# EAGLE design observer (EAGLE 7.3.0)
AUTHOR: B. Campbell, N. Jackson, C. Kreng, A. Zhen; REV: D; TITLE: Observer

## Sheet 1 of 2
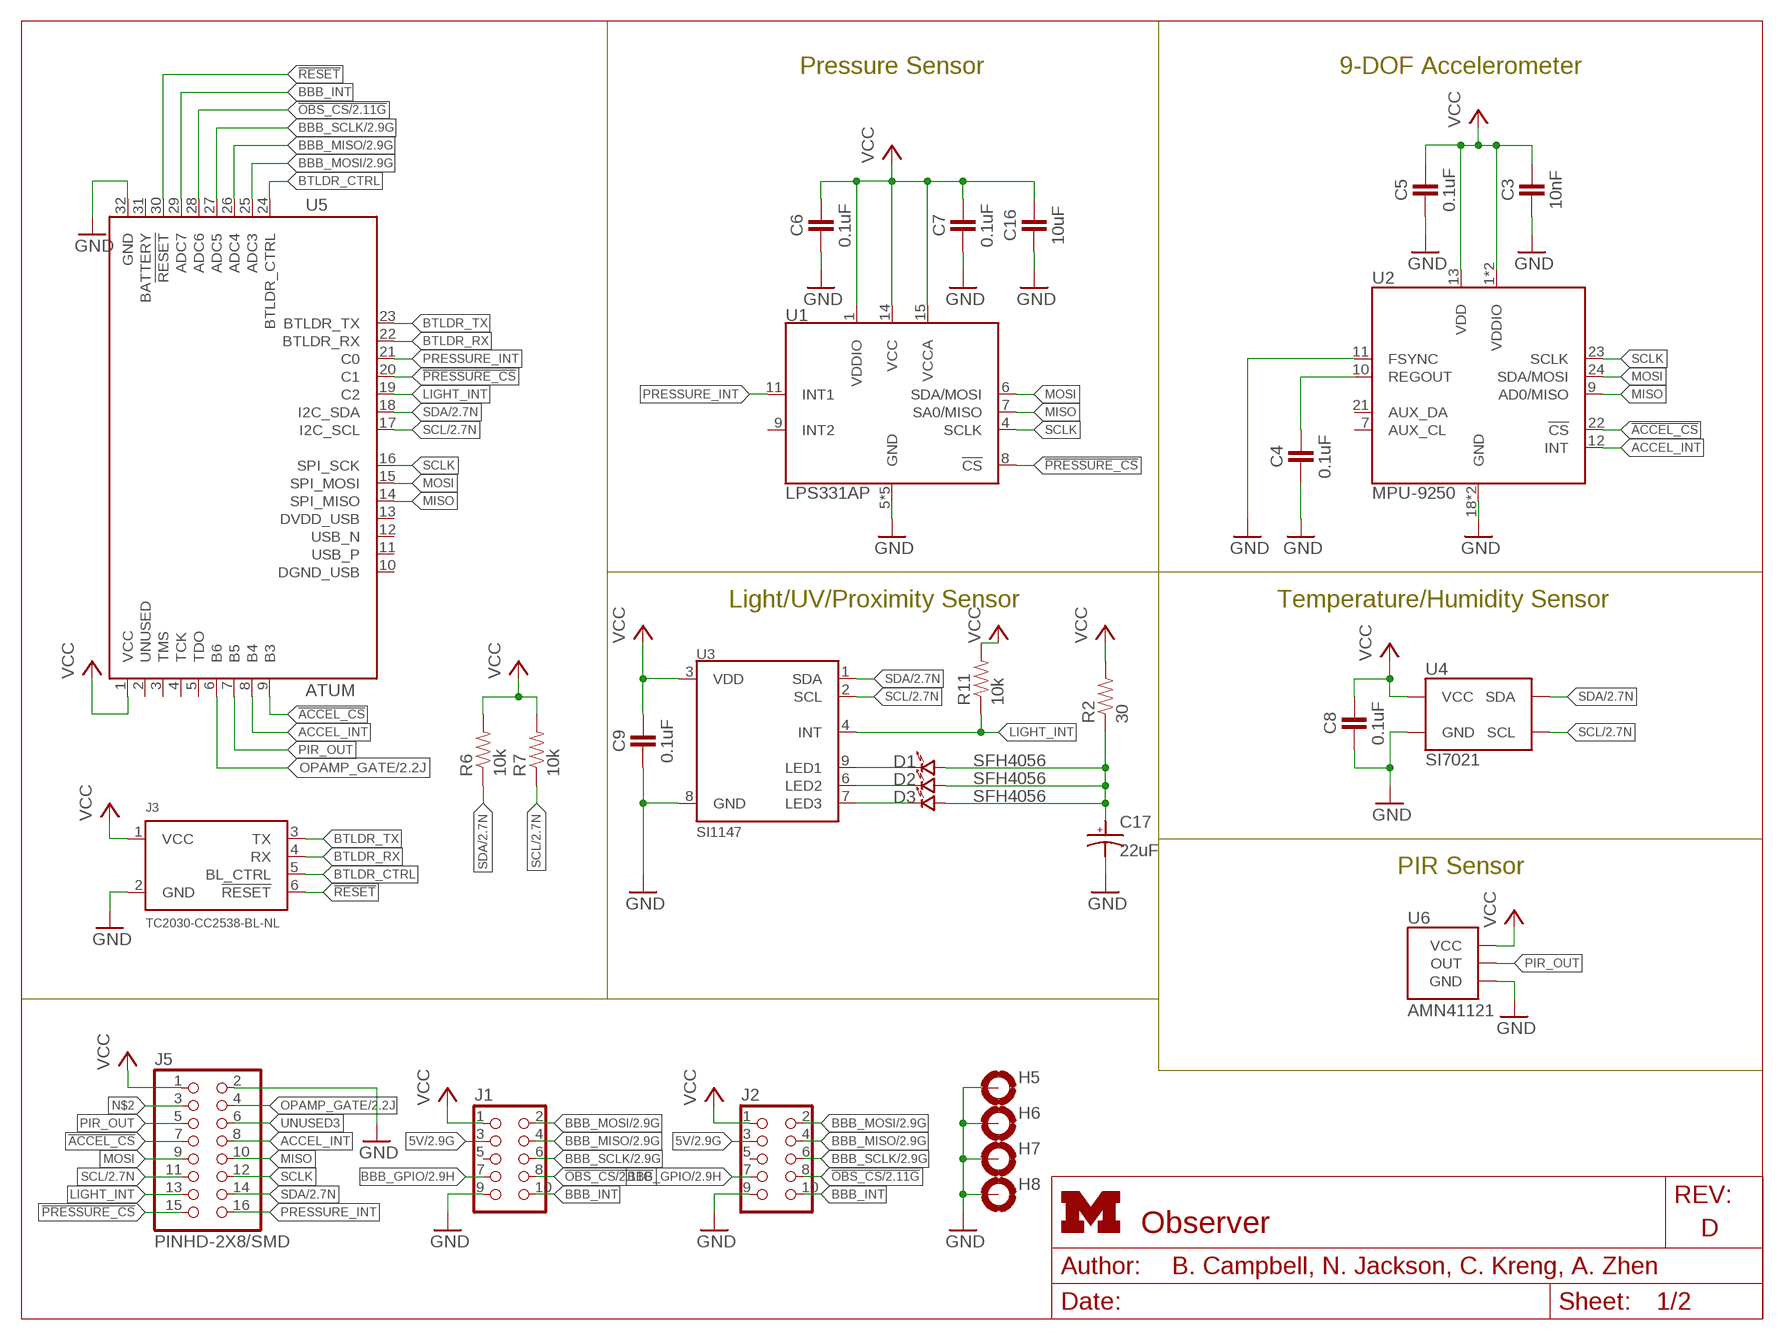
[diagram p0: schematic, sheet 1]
FRAME1 (LETTER_L): HEIGHT: 8.5in; WIDTH: 11in

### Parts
C3  10nF  CAPACITOR  [0402_CAP]
C4  0.1uF  CAPACITOR  [0402_CAP]
C5  0.1uF  CAPACITOR  [0402_CAP]
C6  0.1uF  CAPACITOR  [0402_CAP]
C7  0.1uF  CAPACITOR  [0402_CAP]
C8  0.1uF  CAPACITOR  [0402_CAP]
C9  0.1uF  CAPACITOR  [0402_CAP]
C16  10uF  CAPACITOR  [0402_CAP]
C17  22uF  CAP_POL0603  [CAP0603]
D1  SFH4056  [SFH4056]
D2  SFH4056  [SFH4056]
D3  SFH4056  [SFH4056]
H5  MOUNT-PAD-ROUND3.2  [3,2-PAD]
H6  MOUNT-PAD-ROUND3.2  [3,2-PAD]
H7  MOUNT-PAD-ROUND3.2  [3,2-PAD]
H8  MOUNT-PAD-ROUND3.2  [3,2-PAD]
J1  CON_HEADER_2X05-SMD+SHROUDED  [PINSHRD_SMT_2X05]
J2  CON_HEADER_2X05-SMD+SHROUDED  [PINSHRD_SMT_2X05]
J3  TC2030-CC2538-BL-NL  [TC2030-IDC-NL]
J5  PINHD-2X8/SMD  [2X8/SMD]
R2  30  RESISTOR0402_RES  [0402_RES]
R6  10k  RESISTOR0402_RES  [0402_RES]
R7  10k  RESISTOR0402_RES  [0402_RES]
R11  10k  RESISTOR0402_RES  [0402_RES]
U1  LPS331AP  [HCLGA-16/3MM]
U2  MPU-9250  [QFN-24/3MM]
U3  SI1147  [QFN-10/2MM]
U4  SI7021  [DFN-6/3MM]
U5  ATUM  [ATUM]
U6  AMN41121  [AMN2]

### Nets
5V: J1.3 J2.3 ; also sheet 2
!ACCEL_CS: J5.7 U2.22(!CS) U5.9(B3)
!OBS_CS: J1.8 J2.8 U5.28(ADC6) ; also sheet 2
!PRESSURE_CS: J5.15 U1.8(!CS) U5.20(C1)
!RESET: J3.6(!RESET) U5.30(!RESET)
ACCEL_INT: J5.8 U2.12(INT) U5.8(B4)
BBB_GPIO: J1.7 J2.7 ; also sheet 2
BBB_INT: J1.10 J2.10 U5.29(ADC7)
BBB_MISO: J1.4 J2.4 U5.26(ADC4) ; also sheet 2
BBB_MOSI: J1.2 J2.2 U5.25(ADC3) ; also sheet 2
BBB_SCLK: J1.6 J2.6 U5.27(ADC5) ; also sheet 2
BTLDR_CTRL: J3.5(BL_CTRL) U5.24(BTLDR_CTRL)
BTLDR_RX: J3.4(RX) U5.22(BTLDR_RX)
BTLDR_TX: J3.3(TX) U5.23(BTLDR_TX)
GND: C3.2 C4.2 C5.2 C6.2 C7.2 C8.2 C9.2 C16.2 C17.NEG(ANODE) H5.B3,2(MOUNT) H6.B3,2(MOUNT) H7.B3,2(MOUNT) H8.B3,2(MOUNT) J1.9 J2.9 J3.2(GND) J5.2 U1.5(GND) U1.10(GND) U1.12(GND) U1.13(GND) U1.16(GND) U2.11(FSYNC) U2.18(GND) U2.20(GND) U3.8(GND) U4.2(GND) U5.32(GND) U6.GND ; also sheet 2
LIGHT_INT: J5.13 R11.1 U3.4(INT) U5.19(C2)
MISO: J5.10 U1.7(SA0/MISO) U2.9(AD0/MISO) U5.14(SPI_MISO)
MOSI: J5.9 U1.6(SDA/MOSI) U2.24(SDA/MOSI) U5.15(SPI_MOSI)
N$2: J5.3
N$3: C4.1 U2.10(REGOUT)
N$4: D1.CATHODE U3.9(LED1)
N$6: D2.CATHODE U3.6(LED2)
N$7: D3.CATHODE U3.7(LED3)
N$8: C17.POS(CATHODE) D1.ANODE D2.ANODE D3.ANODE R2.1
OPAMP_GATE: J5.4 U5.6(B6) ; also sheet 2
PIR_OUT: J5.5 U5.7(B5) U6.OUT
PRESSURE_INT: J5.16 U1.11(INT1) U5.21(C0)
SCL: J5.11 R7.1 U3.2(SCL) U4.6(SCL) U5.17(I2C_SCL) ; also sheet 2
SCLK: J5.12 U1.4(SCLK) U2.23(SCLK) U5.16(SPI_SCK)
SDA: J5.14 R6.1 U3.1(SDA) U4.1(SDA) U5.18(I2C_SDA) ; also sheet 2
UNUSED3: J5.6
VCC: C3.1 C5.1 C6.1 C7.1 C8.1 C9.1 C16.1 J1.1 J2.1 J3.1(VCC) J5.1 R2.2 R6.2 R7.2 R11.2 U1.1(VDDIO) U1.14(VCC) U1.15(VCCA) U2.1(VDDIO) U2.8(VDDIO) U2.13(VDD) U3.3(VDD) U4.5(VCC) U5.1(VCC) U6.VCC ; also sheet 2
Unconnected: J1.5 J2.5 U1.9(INT2) U2.7(AUX_CL) U2.21(AUX_DA) U5.2(UNUSED) U5.3(TMS) U5.4(TCK) U5.5(TDO) U5.10(DGND_USB) U5.11(USB_P) U5.12(USB_N) U5.13(DVDD_USB) U5.31(BATTERY)

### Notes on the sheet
- Pressure Sensor | 9-DOF Accelerometer
- Light/UV/Proximity Sensor | Temperature/Humidity Sensor
- PIR Sensor

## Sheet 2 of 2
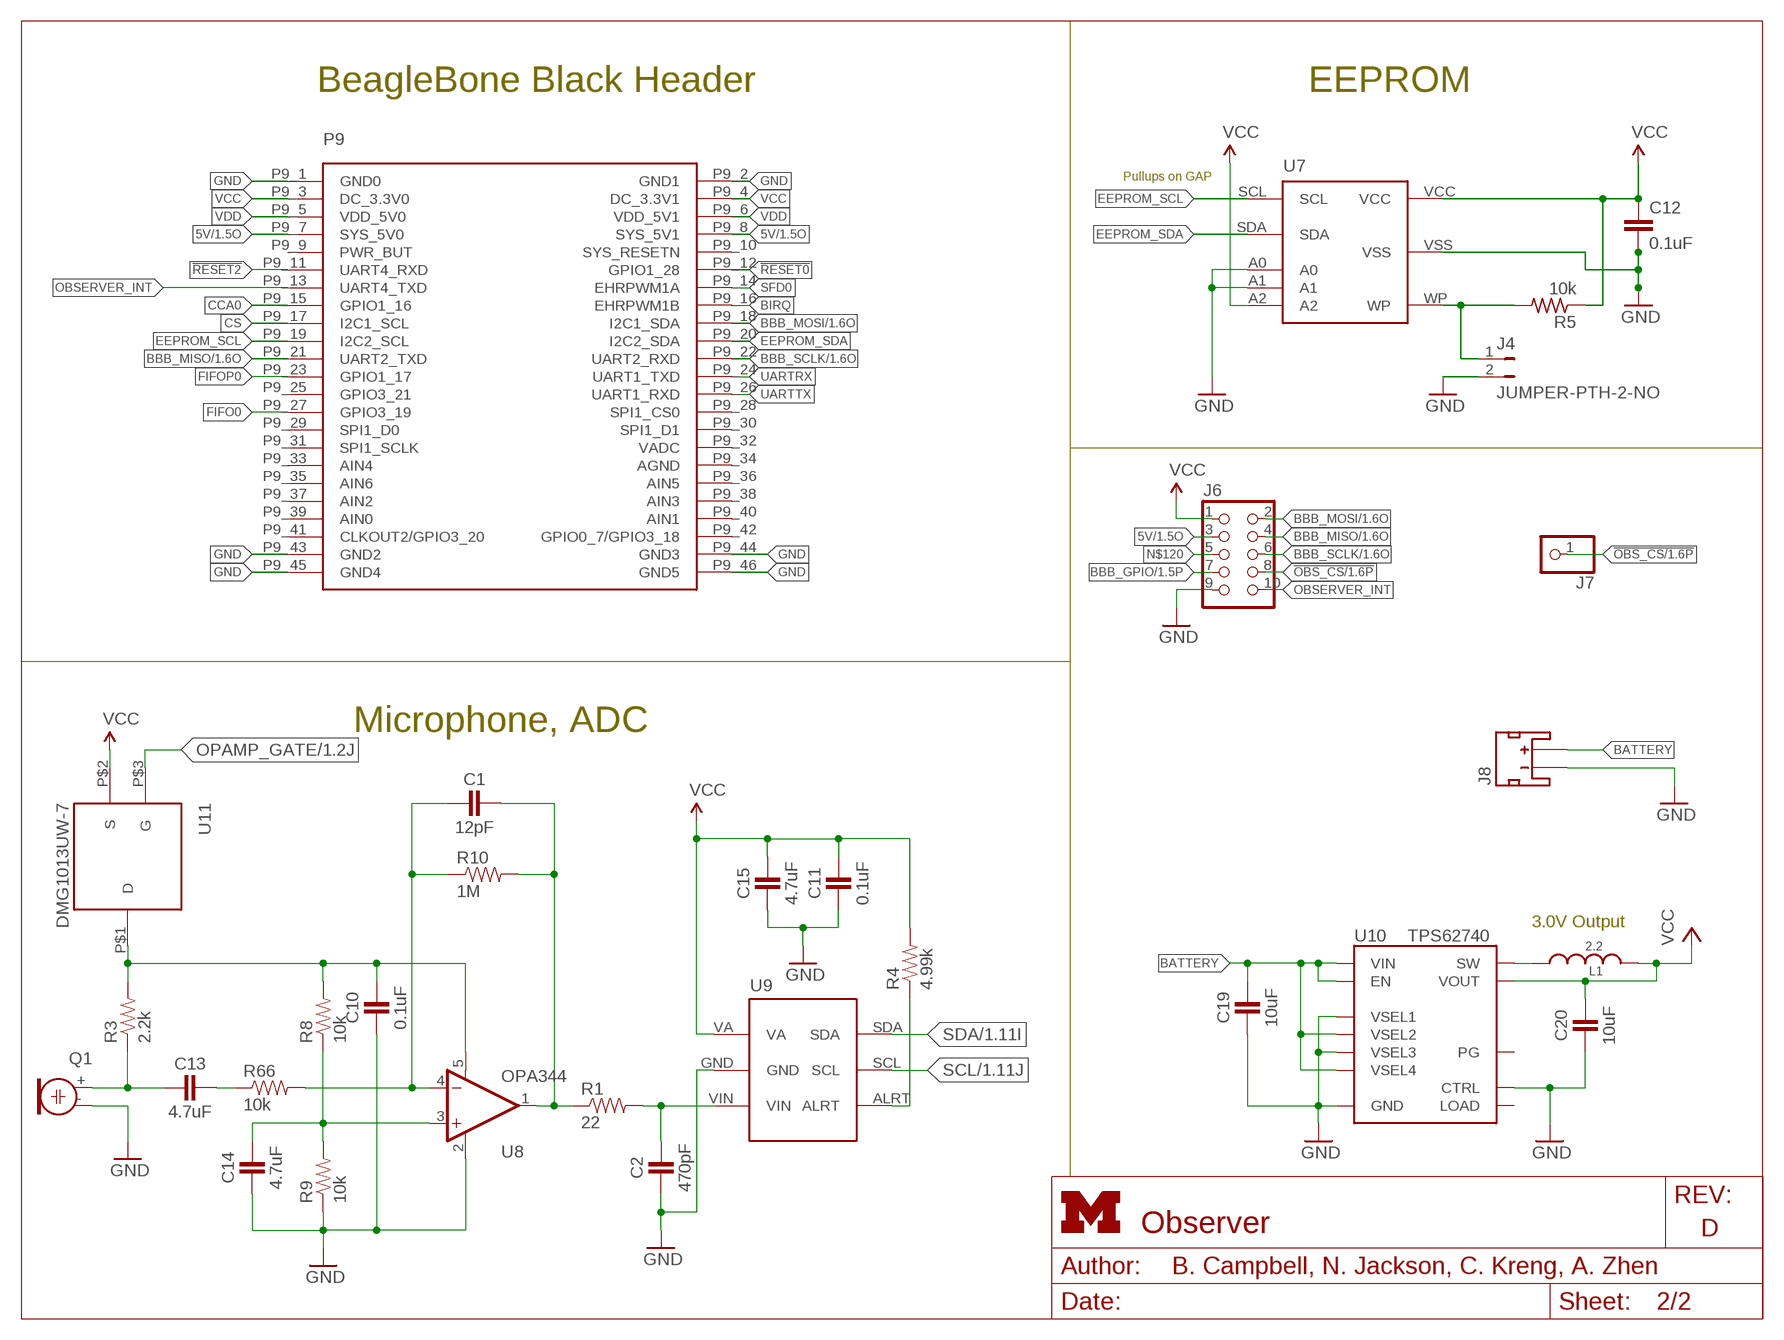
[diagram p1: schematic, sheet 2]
FRAME2 (LETTER_L): HEIGHT: 8.5in; WIDTH: 11in

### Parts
C1  12pF  CAPACITOR  [0402_CAP]
C2  470pF  CAPACITOR  [0402_CAP]
C10  0.1uF  CAPACITOR  [0402_CAP]
C11  0.1uF  CAPACITOR  [0402_CAP]
C12  0.1uF  C-EUC0402  [C0402]
C13  4.7uF  CAPACITOR  [0402_CAP]
C14  4.7uF  CAPACITOR  [0402_CAP]
C15  4.7uF  CAPACITOR  [0402_CAP]
C19  10uF  CAPACITOR0603_CAP  [0603_CAP]
C20  10uF  CAPACITOR0603_CAP  [0603_CAP]
J4  JUMPER-PTH-2-NO  [PTH-JUMPER-2-NO_NO_SILK]
J6  CON_HEADER_2X05-PTH+SHROUDED_A  [PINSHRD_PTH_2X05]
J7  PINHD-1X1  [1X01]
J8  JST_2MM_MALE  [JST-2-SMD]
L1  2.2  MIPSZ2012D  [MIPSZ201D]
P9/P8  BBB_HEADER  [BBB_HEADERS]
Q1  ELECTRET  [ELECTRET_9.7]
R1  22  RESISTOR0402_RES  [0402_RES]
R3  2.2k  RESISTOR0402_RES  [0402_RES]
R4  4.99k  RESISTOR0402_RES  [0402_RES]
R5  10k  R-US_R0402  [R0402]
R8  10k  RESISTOR0402_RES  [0402_RES]
R9  10k  RESISTOR0402_RES  [0402_RES]
R10  1M  RESISTOR0402_RES  [0402_RES]
R66  10k  RESISTOR0402_RES  [0402_RES]
U7  CAT24C256WI-GT3  [CAT24C256WI-GT3]
U8  OPA344  [SOT23-5]
U9  ADC121C021  [ADC121C021]
U10  TPS62740  [R-PWSON-12]
U11  DMG1013UW-7  [SOT-323]

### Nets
5V: J6.3 P9/P8.P9_7(SYS_5V0) P9/P8.P9_8(SYS_5V1) ; also sheet 1
!OBS_CS: J6.8 J7.1 ; also sheet 1
!RESET0: P9/P8.P9_12(GPIO1_28)
!RESET2: P9/P8.P9_11(UART4_RXD)
BATTERY: C19.1 J8.2(+) U10.1(VIN) U10.8(VSEL4) U10.10(VSEL2) U10.12(EN)
BBB_GPIO: J6.7 ; also sheet 1
BBB_MISO: J6.4 P9/P8.P9_21(UART2_TXD) ; also sheet 1
BBB_MOSI: J6.2 P9/P8.P9_18(I2C1_SDA) ; also sheet 1
BBB_SCLK: J6.6 P9/P8.P9_22(UART2_RXD) ; also sheet 1
BIRQ: P9/P8.P9_16(EHRPWM1B)
CCA0: P9/P8.P9_15(GPIO1_16)
CS: P9/P8.P9_17(I2C1_SCL)
EEPROM_SCL: P9/P8.P9_19(I2C2_SCL) U7.SCL
EEPROM_SDA: P9/P8.P9_20(I2C2_SDA) U7.SDA
FIFO0: P9/P8.P9_27(GPIO3_19)
FIFOP0: P9/P8.P9_23(GPIO1_17)
GND: C2.2 C10.2 C11.2 C12.2 C14.2 C15.2 C19.2 C20.2 J4.2 J6.9 J8.1(-) P9/P8.P9_1(GND0) P9/P8.P9_2(GND1) P9/P8.P9_43(GND2) P9/P8.P9_44(GND3) P9/P8.P9_45(GND4) P9/P8.P9_46(GND5) Q1.- R9.1 U7.A0 U7.A1 U7.VSS U8.2(V-) U9.GND U10.3(GND) U10.4(CTRL) U10.9(VSEL3) U10.11(VSEL1) U10.NC(GND) ; also sheet 1
MIC_AIN: C1.1 R1.1 R10.2 U8.1(OUT)
MIC_INT: R4.1 U9.ALRT
N$1: C13.2 Q1.+ R3.1
N$5: C13.1 R66.1
N$9: C1.2 R10.1 R66.2 U8.4(-IN)
N$10: C14.1 R8.1 R9.2 U8.3(+IN)
N$11: C2.1 R1.2 U9.VIN
N$12: L1.1 U10.2(SW)
N$14: C10.1 R3.2 R8.2 U8.5(V+) U11.P$1(D)
N$31: J4.1 R5.2 U7.WP
N$120: J6.5
OBSERVER_INT: J6.10 P9/P8.P9_13(UART4_TXD)
OPAMP_GATE: U11.P$3(G) ; also sheet 1
SCL: U9.SCL ; also sheet 1
SDA: U9.SDA ; also sheet 1
SFD0: P9/P8.P9_14(EHRPWM1A)
UARTRX: P9/P8.P9_24(UART1_TXD)
UARTTX: P9/P8.P9_26(UART1_RXD)
VCC: C11.1 C12.1 C15.1 C20.1 J6.1 L1.2 P9/P8.P9_3(DC_3.3V0) P9/P8.P9_4(DC_3.3V1) R4.2 R5.1 U7.A2 U7.VCC U9.VA U10.5(VOUT) U11.P$2(S) ; also sheet 1
VDD: P9/P8.P9_5(VDD_5V0) P9/P8.P9_6(VDD_5V1)
Unconnected: J8.NC1(PAD1) J8.NC2(PAD2) P9/P8.P9_9(PWR_BUT) P9/P8.P9_10(SYS_RESETN) P9/P8.P9_25(GPIO3_21) P9/P8.P9_28(SPI1_CS0) P9/P8.P9_29(SPI1_D0) P9/P8.P9_30(SPI1_D1) P9/P8.P9_31(SPI1_SCLK) P9/P8.P9_32(VADC) P9/P8.P9_33(AIN4) P9/P8.P9_34(AGND) P9/P8.P9_35(AIN6) P9/P8.P9_36(AIN5) P9/P8.P9_37(AIN2) P9/P8.P9_38(AIN3) P9/P8.P9_39(AIN0) P9/P8.P9_40(AIN1) P9/P8.P9_41(CLKOUT2/GPIO3_20) P9/P8.P9_42(GPIO0_7/GPIO3_18) U10.6(LOAD) U10.7(PG)

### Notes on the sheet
- BeagleBone Black Header | EEPROM
- Pullups on GAP
- Microphone, ADC
- 3.0V Output

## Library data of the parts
C1 C2 C10 C11 C13-C15 = passives:CAPACITOR: 0402 Capacitor
C3 = passives:CAPACITOR: 0402 Capacitor; DIGIKEY: 490-1312-1-ND
C4-C9 = passives:CAPACITOR: 0402 Capacitor; DIGIKEY: 490-1318-1-ND
C12 = rcl:C-EU: CAPACITOR, European symbol; DIGIKEY: 490-1318-1-ND
C16 = passives:CAPACITOR: 0402 Capacitor; DIGIKEY: 445-8919-1-ND
C17 = passives:CAP_POL; DIGIKEY: 511-1493-1-ND
C19 C20 = passives:CAPACITOR: 0402 Capacitor; DIGIKEY: 490-7316-1-ND
D1-D3 = leds:SFH4056: LED IR EMITTER 850NM; DIGIKEY: 475-3042-1-ND
H5-H8 = holes:MOUNT-PAD-ROUND: MOUNTING PAD, round
J1 J2 = dp_devices:CON_HEADER_2X05: 2x05 pin header; DIGIKEY: S9185-ND
J3 = connector:TC2030-CC2538-BL: Tag connect programmer for the CC2538 bootloader. The RX/TX switch happens on the programmer board, so when using this connect the TX pin to the TX pin on the CC2538 and same for the RX.
J4 = SparkFun-Passives:JUMPER-PTH-2-NO
J5 = headers:PINHD-2X8/SMD
J6 = dp_devices:CON_HEADER_2X05: 2x05 pin header
J7 = pinhead:PINHD-1X1: PIN HEADER
J8 = SparkFun-Connectors:JST_2MM_MALE: Mates to single-cell LiPo batteries. CONN-11443 Now with smashable polarity marks!; BTM_NEG: -; BTM_POS: +; PROD_ID: CONN-11443; TOP_NEG: -; TOP_POS: +
L1 = passives:MIPSZ2012D: FDK Multi-layer Power Inductor : MIPSZ2012D series (Very Small Type)
P9/P8 = observer:BBB_HEADER: Beaglebone Black P9 Pin Header 2x23
Q1 = observer:ELECTRET: Electret microphone
R1 R3 R4 R8-R10 R66 = passives:RESISTOR: Resistor
R2 R11 = passives:RESISTOR: Resistor; DIGIKEY: RHM30CECT-ND
R5 = rcl:R-US_: RESISTOR, American symbol; DIGIKEY: RHM1.00MCDCT-ND
R6 R7 = passives:RESISTOR: Resistor; DIGIKEY: RHM10.0KCDCT-ND
U1 = chips:LPS331AP: IC PRESSURE SENSOR PIEZO 16HCLGA; DIGIKEY: 497-12927-1-ND
U2 = chips:MPU-9250: GYRO/ACCEL/COMPASS/9-AXIS; DIGIKEY: 1428-1019-1-ND
U3 = chips:SI1147: SENSOR DGTL UV INDEX 10QFN; DIGIKEY: 336-2624-1-ND
U4 = chips:SI7021: IC TEMP SENSOR RH 2% DFN; DIGIKEY: 336-2542-1-ND
U5 = atum:ATUM: Atum sensorboard prototyping module.
U6 = chips:AMN: Passive infrared human detection sensor with built-in amp.; DIGIKEY: 255-2651-ND
U7 = bbb-cc2520:CAT24C256: 256kb Serial CMOS EEPROM, organized as 32,768 words of 8 bits each
U8 = SparkFun-AnalogIC:OPA344: Single gate rail-to-rail output op-amp. Inputs extend 300mV past rails.
U9 = observer:ADC121C021
U10 = chips:TPS62740: 360nA Step Down Converter for Low Power Applications; DIGIKEY: 296-37134-1-ND; MOUSER: 595-TPS62740DSST; NEWARK: 27X9745
U11 = pfet:DMG1013UW-7

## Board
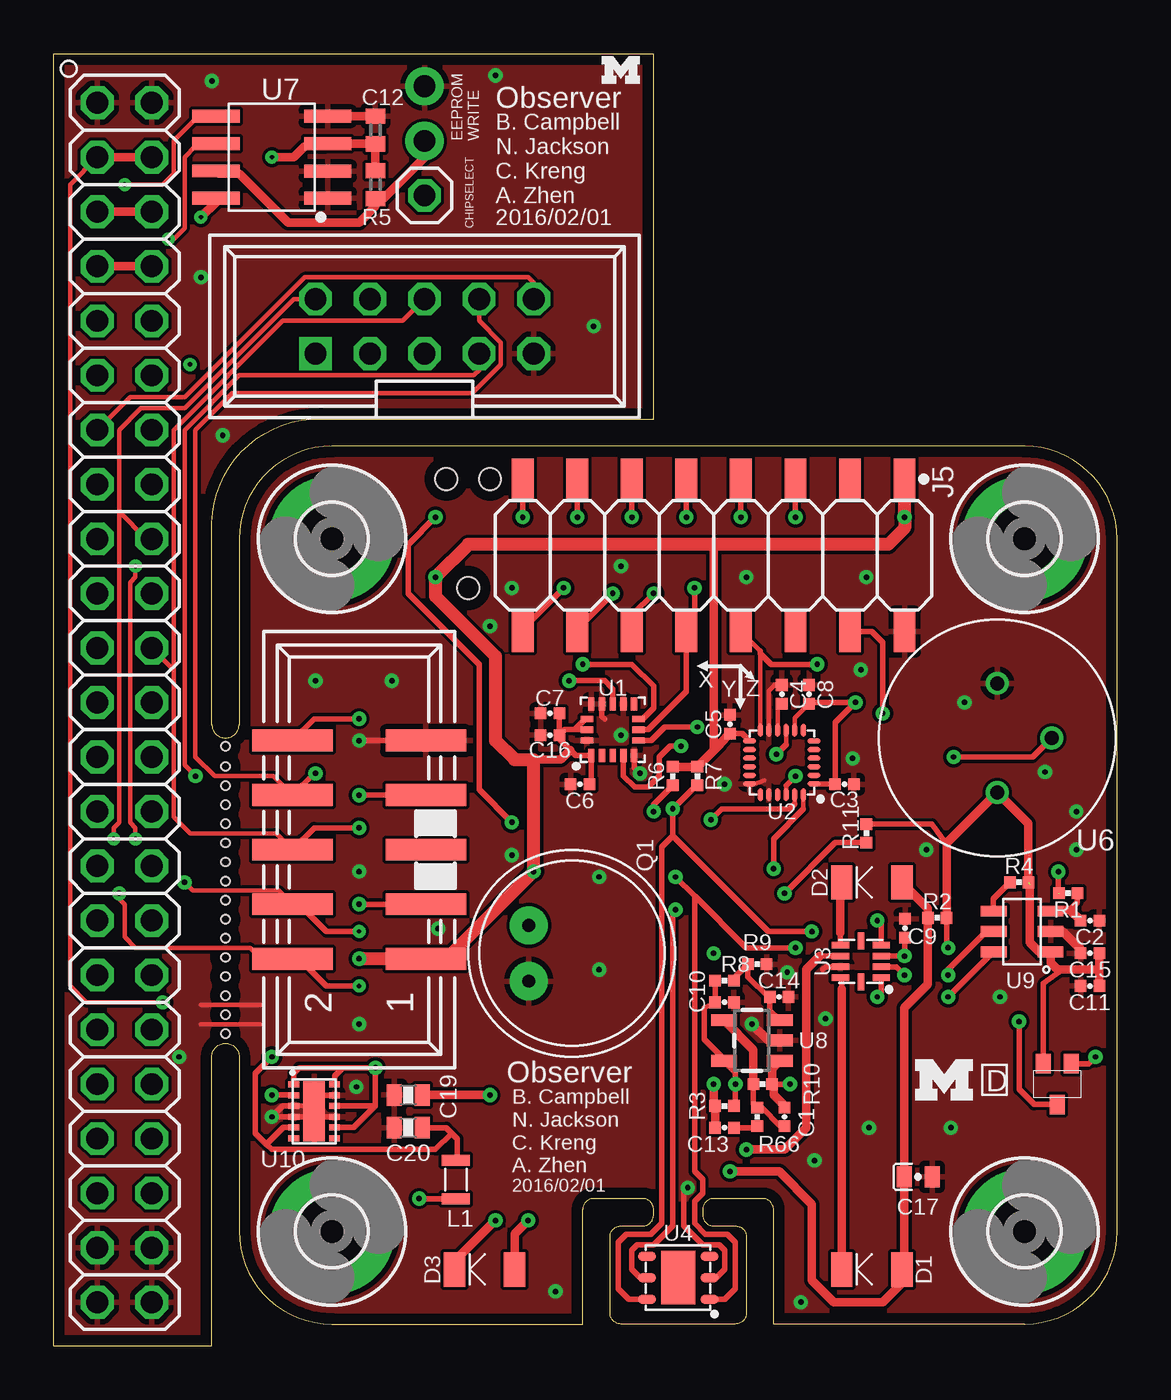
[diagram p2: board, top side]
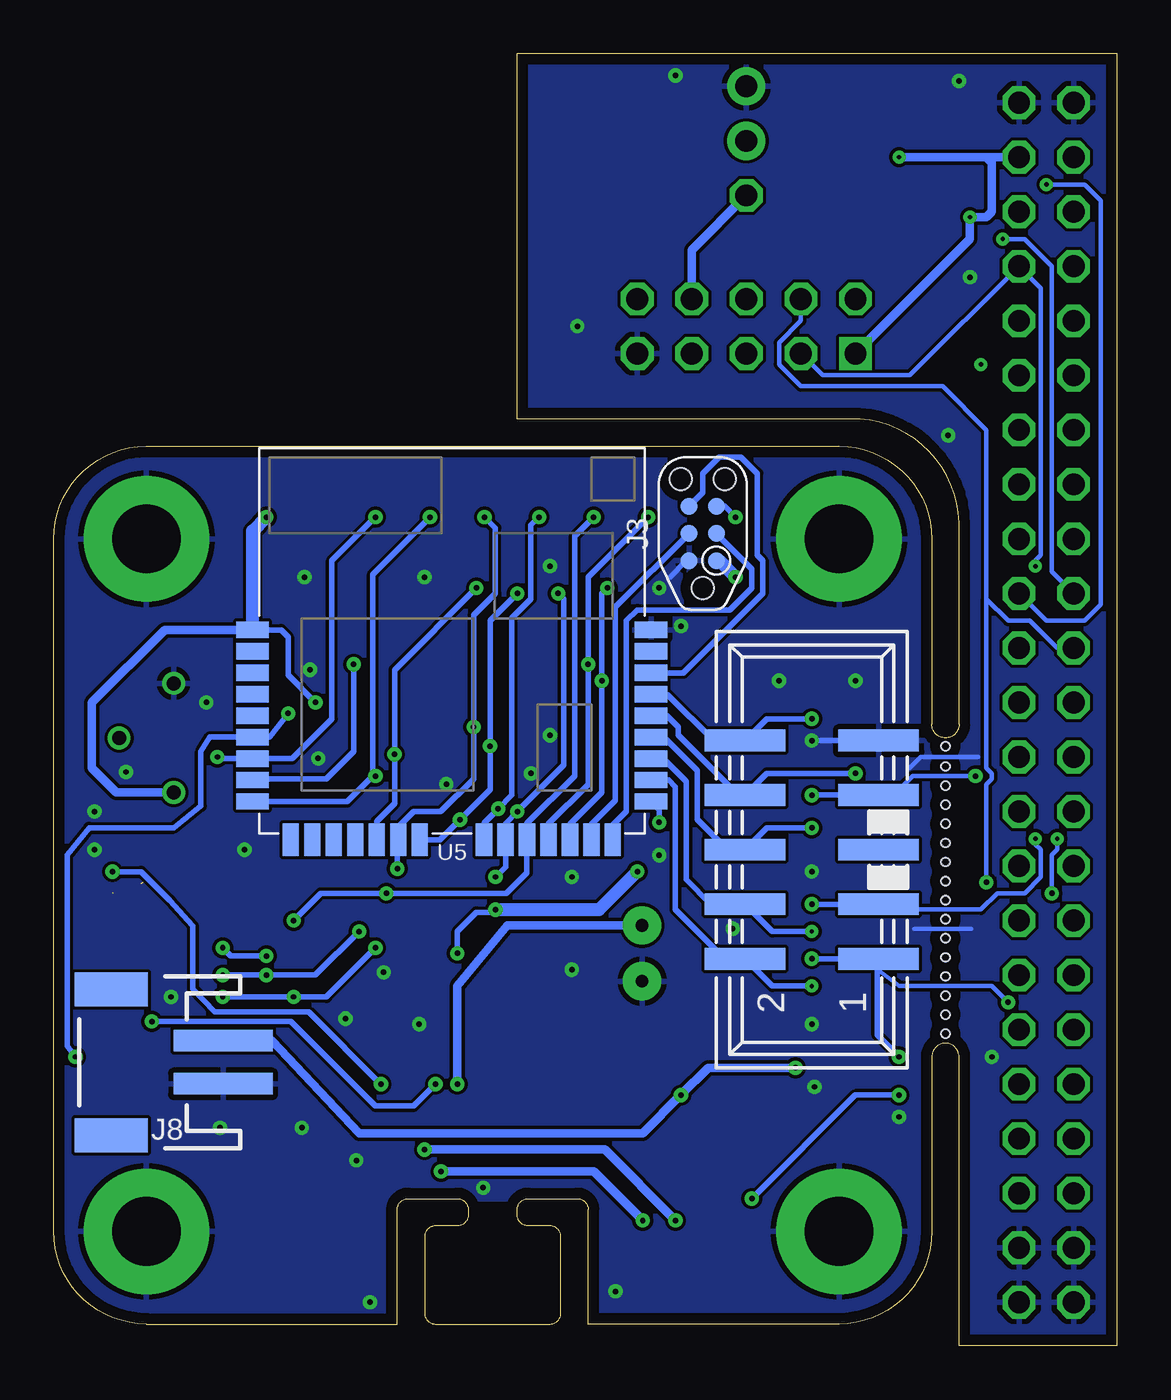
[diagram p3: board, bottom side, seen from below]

Size 49.53 x 60.2 mm. Coordinates in mm from the lower left corner, seen from the top.
Outline: 49.53,5.33 49.53,37.59 arc90 45.21,41.91 12.95,41.91 arc90 8.64,37.59 8.64,28.96 arc-180 7.37,28.96 7.37,38.35 arc-90 12.45,43.18 27.94,43.18 27.94,60.2 0,60.2 0,0 7.37,0 7.37,13.46 arc-180 8.64,13.46 8.64,5.33 arc90 12.95,1.02 24.64,1.02 24.64,6.35 arc-90 25.15,6.86 27.43,6.86 arc-90 27.94,6.35 27.94,6.1 arc-90 27.43,5.59 26.42,5.59 arc90 25.91,5.08 25.91,1.52 arc90 26.42,1.02 31.75,1.02 arc90 32.26,1.52 32.26,5.08 arc90 31.75,5.59 30.73,5.59 arc-90 30.23,6.1 30.23,6.35 arc-90 30.73,6.86 33.02,6.86 arc-90 33.53,6.35 33.53,1.02 45.21,1.02 arc90 49.53,5.33
Copper layers (1*16): Top 0.0178mm / dielectric 59mil / Bottom 0.0178mm
Design rules "sunstone-2lyr_v1.0.0.3 *": minimum track width 6mil, minimum drill 8mil, track to track 6mil, track to pad 6mil, pad to pad 6mil, via to via 6mil, smd to smd 6mil, copper to edge 20mil, drill to drill 16mil, minimum pad ring 8mil, minimum via ring 8mil, stop-mask expansion 3mil, vias tented up to drill 50mil, thermal gap 10mil
Holes 0.38 mm at 8,26.99 8,26.1 8,25.21 8,24.32 8,23.43 8,22.54 8,21.65 8,20.76 8,19.88 8,18.99 8,18.1 8,17.21 8,16.32 8,15.43 8,14.54 8,27.94

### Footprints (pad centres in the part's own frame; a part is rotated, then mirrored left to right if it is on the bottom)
0402_CAP = smd 0.536 x 0.546: 1 -0.433,0; 2 0.433,0
C0402 = smd 0.7 x 0.9: 1 -0.65,0; 2 0.65,0
CAP0603 = smd 0.7 x 1: NEG 0.65,0; POS -0.65,0
0603_CAP = smd 0.7 x 1: 1 -0.65,0; 2 0.65,0
SFH4056 = smd 1 x 1.6: ANODE 1.4,0; CATHODE -1.4,0
3,2-PAD = drill 3.2 pad 5.842: B3,2 0,0
PINSHRD_SMT_2X05 = smd 1.02 x 3.75: 1 -5.08,-3.107; 2 -5.08,3.107; 3 -2.54,-3.107; 4 -2.54,3.107; 5 0,-3.107; 6 0,3.107; 7 2.54,-3.107; 8 2.54,3.107; 9 5.08,-3.107; 10 5.08,3.107
TC2030-IDC-NL = smd 0.787 x 0.787: 1 -1.27,-0.635; 2 -1.27,0.635; 3 0,-0.635; 4 0,0.635; 5 1.27,-0.635; 6 1.27,0.635 | hole 1.016: -2.54,0; 2.54,1.016; 2.54,-1.016
PTH-JUMPER-2-NO_NO_SILK = drill 1.016 pad 1.778: 1 -1.27,0; 2 1.27,0
2X8/SMD = smd 1.016 x 1.905: 1 -8.89,-3.556; 2 -8.89,3.556; 3 -6.35,-3.556; 4 -6.35,3.556; 5 -3.81,-3.556; 6 -3.81,3.556; 7 -1.27,-3.556; 8 -1.27,3.556; 9 1.27,-3.556; 10 1.27,3.556; 11 3.81,-3.556; 12 3.81,3.556; 13 6.35,-3.556; 14 6.35,3.556; 15 8.89,-3.556; 16 8.89,3.556
PINSHRD_PTH_2X05 = drill 1.016 square: 1 -5.08,-1.27 | drill 1.016 octagon: 2 -5.08,1.27; 3 -2.54,-1.27; 4 -2.54,1.27; 5 0,-1.27; 6 0,1.27; 7 2.54,-1.27; 8 2.54,1.27; 9 5.08,-1.27; 10 5.08,1.27
1X01 = drill 1.016 octagon: 1 0,0
JST-2-SMD = smd 1 x 4.6: 1 -1,-3.7; 2 1,-3.7 | smd 1.6 x 3.4: NC1 -3.4,1.5; NC2 3.4,1.5
MIPSZ201D = smd 0.5 x 1.3: 1 -0.9,0; 2 0.9,0
BBB_HEADERS = drill 1.016 octagon: P9_1 1.27,57.15; P9_2 3.81,57.15; P9_3 1.27,54.61; P9_4 3.81,54.61; P9_5 1.27,52.07; P9_6 3.81,52.07; P9_7 1.27,49.53; P9_8 3.81,49.53; P9_9 1.27,46.99; P9_10 3.81,46.99; P9_11 1.27,44.45; P9_12 3.81,44.45; P9_13 1.27,41.91; P9_14 3.81,41.91; P9_15 1.27,39.37; P9_16 3.81,39.37; P9_17 1.27,36.83; P9_18 3.81,36.83; P9_19 1.27,34.29; P9_20 3.81,34.29; P9_21 1.27,31.75; P9_22 3.81,31.75; P9_23 1.27,29.21; P9_24 3.81,29.21; P9_25 1.27,26.67; P9_26 3.81,26.67; P9_27 1.27,24.13; P9_28 3.81,24.13; P9_29 1.27,21.59; P9_30 3.81,21.59; P9_31 1.27,19.05; P9_32 3.81,19.05; P9_33 1.27,16.51; P9_34 3.81,16.51; P9_35 1.27,13.97; P9_36 3.81,13.97; P9_37 1.27,11.43; P9_38 3.81,11.43; P9_39 1.27,8.89; P9_40 3.81,8.89; P9_41 1.27,6.35; P9_42 3.81,6.35; P9_43 1.27,3.81; P9_44 3.81,3.81; P9_45 1.27,1.27; P9_46 3.81,1.27
ELECTRET_9.7 = drill 0.6 pad 1.778: + 1.3,2; - -1.3,2
0402_RES = smd 0.536 x 0.546: 1 -0.433,0; 2 0.433,0
R0402 = smd 0.7 x 0.9: 1 -0.65,0; 2 0.65,0
HCLGA-16/3MM = smd 0.6 x 0.3: 1 -1.2,1; 2 -1.2,0.5; 3 -1.2,0; 4 -1.2,-0.5; 5 -1.2,-1; 9 1.2,-1; 10 1.2,-0.5; 11 1.2,0; 12 1.2,0.5; 13 1.2,1 | smd 0.3 x 0.6: 6 -0.5,-1.2; 7 0,-1.2; 8 0.5,-1.2; 14 0.5,1.2; 15 0,1.2; 16 -0.5,1.2
QFN-24/3MM = smd 0.6 x 0.23: 1 -1.5,1; 2 -1.5,0.6; 3 -1.5,0.2; 4 -1.5,-0.2; 5 -1.5,-0.6; 6 -1.5,-1; 13 1.5,-1; 14 1.5,-0.6; 15 1.5,-0.2; 16 1.5,0.2; 17 1.5,0.6; 18 1.5,1 | smd 0.23 x 0.6: 7 -1,-1.5; 8 -0.6,-1.5; 9 -0.2,-1.5; 10 0.2,-1.5; 11 0.6,-1.5; 12 1,-1.5; 19 1,1.5; 20 0.6,1.5; 21 0.2,1.5; 22 -0.2,1.5; 23 -0.6,1.5; 24 -1,1.5
QFN-10/2MM = smd 0.8 x 0.3: 1 -0.95,0.75; 2 -0.95,0.25; 3 -0.95,-0.25; 4 -0.95,-0.75; 6 0.95,-0.75; 7 0.95,-0.25; 8 0.95,0.25; 9 0.95,0.75 | smd 0.3 x 0.8: 5 0,-0.95; 10 0,0.95
DFN-6/3MM = smd 0.85 x 0.45: 1 -1.45,1; 2 -1.45,0; 3 -1.45,-1; 4 1.45,-1; 5 1.45,0; 6 1.45,1 | smd 1.6 x 2.5: P$1 0,0
ATUM = smd 0.754 x 1.5: 1 -9.479,-9.279; 2 -8.479,-9.279; 3 -7.479,-9.279; 4 -6.479,-9.279; 5 -5.479,-9.279; 6 -4.479,-9.279; 7 -3.479,-9.279; 8 -2.479,-9.279; 9 -1.479,-9.279; 24 -1.479,9.279; 25 -2.479,9.279; 26 -3.479,9.279; 27 -4.479,9.279; 28 -5.479,9.279; 29 -6.479,9.279; 30 -7.479,9.279; 31 -8.479,9.279; 32 -9.479,9.279 | smd 1.5 x 0.754: 10 0.3,-7.5; 11 0.3,-6.5; 12 0.3,-5.5; 13 0.3,-4.5; 14 0.3,-3.5; 15 0.3,-2.5; 16 0.3,-1.5; 17 0.3,1.5; 18 0.3,2.5; 19 0.3,3.5; 20 0.3,4.5; 21 0.3,5.5; 22 0.3,6.5; 23 0.3,7.5
AMN2 = drill 0.65: GND 1.796,-1.796; OUT -1.796,-1.796; VCC -1.796,1.796
CAT24C256WI-GT3 = smd 2.2 x 0.6: A0 -2.6,1.91; A1 -2.6,0.65; A2 -2.6,-0.64; SCL 2.6,-0.64; SDA 2.6,-1.91; VCC 2.6,1.91; VSS -2.6,-1.91; WP 2.6,0.64
SOT23-5 = smd 0.55 x 1.2: 1 -0.95,-1.3; 2 0,-1.3; 3 0.95,-1.3; 4 0.95,1.3; 5 -0.95,1.3
ADC121C021 = smd 1.2 x 0.5: ALRT 2.2,0.575; GND -0.45,1.525; SCL 2.2,1.525; SDA 2.2,2.475; VA -0.45,2.475; VIN -0.45,0.575
R-PWSON-12 = smd 0.28 x 0.5: 1 -1.25,-0.95; 2 -0.75,-0.95; 3 -0.25,-0.95; 4 0.25,-0.95; 5 0.75,-0.95; 6 1.25,-0.95; 7 1.25,0.95; 8 0.75,0.95; 9 0.25,0.95; 10 -0.25,0.95; 11 -0.75,0.95; 12 -1.25,0.95 | smd 2.8 x 1: NC 0,0
SOT-323 = smd 0.7 x 0.9: P$1 0,0.95; P$2 0.65,-0.95; P$3 -0.65,-0.95

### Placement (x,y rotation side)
C1  34.04,10.67 270 top
C2  48.26,19.81 0 top
C3  36.83,26.16 0 top
C4  33.91,30.35 90 top
C5  31.5,28.96 90 top
C6  24.51,26.16 180 top
C7  23.11,29.46 180 top
C8  35.18,30.35 90 top
C9  39.65,19.46 90 top
C10  31.24,16 0 top
C11  48.26,16.76 180 top
C12  14.99,56.64 90 top
C13  31.24,10.16 180 top
C14  33.78,16.26 0 top
C15  48.26,18.29 180 top
C16  23.11,28.45 180 top
C17  40.26,7.87 0 top
C19  16.51,11.68 180 top
C20  16.51,10.16 180 top
D1  38.1,3.56 0 top
D2  38.1,21.59 0 top
D3  20.07,3.56 0 top
H5  45.21,37.59 180 top
H6  45.21,5.33 180 top
H7  12.95,5.33 180 top
H8  12.95,37.59 0 top
J1  14.22,23.11 90 bottom
J2  14.22,23.11 90 top
J3  19.3,37.85 90 bottom
J4  17.27,57.4 90 top
J5  30.73,36.83 180 top
J6  17.27,47.5 0 top
J7  17.27,53.59 0 top
J8  45.34,13.21 90 bottom
L1  18.73,7.75 90 top
P9/P8  0.76,0.76 0 top
Q1  24.13,18.29 90 top
R1  47.24,21.08 0 top
R2  41.15,19.94 0 top
R3  31.24,11.18 0 top
R4  44.96,21.59 0 top
R5  14.99,54.1 270 top
R6  28.83,26.54 90 top
R7  29.97,26.54 90 top
R8  31.24,17.02 180 top
R9  32.77,17.78 180 top
R10  33.02,12.19 0 top
R11  37.85,23.88 90 top
R66  32.77,10.67 90 top
U1  26.04,28.7 90 top
U2  33.91,27.18 180 top
U3  37.59,17.91 180 top
U4  29.08,3.17 180 top
U5  30.99,23.88 270 bottom
U6  43.94,28.32 135 top
U7  10.16,55.37 180 top
U8  32.51,14.22 90 top
U9  45.97,20.83 180 top
U10  12.13,10.92 270 top
U11  46.74,12.19 180 top
U$1  [UMICH_SOLID_75MIL]  40.13,11.43 0 top
U$2  [UMICH_SOLID_50MIL]  26.42,59.44 0 top

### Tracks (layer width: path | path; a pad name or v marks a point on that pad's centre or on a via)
5V  (via drill 0.2, 0.25)
  Top 0.203: v3.81,36.32 3.81,35.81 3.56,35.56 3.56,24.38 3.81,24.13 v3.81,23.62
  Top 0.254: J2.3 v14.22,20.57
  Top 0.406: P9/P8.P9_7 P9/P8.P9_8
  Bottom 0.203: J6.3 13.72,45.21 9.65,45.21 P9/P8.P9_8 3.56,49.28 3.56,36.83 3.81,36.58 v3.81,36.32 | v3.81,23.62 3.81,23.37 3.56,23.11 3.56,21.84 4.32,21.08 5.59,21.08 6.35,20.32 10.03,20.32 10.41,20.7 | J1.3 10.99,20.7 10.41,20.7 | 10.41,20.7 9.53,20.7 9.4,20.57
  Bottom 0.254: v14.22,20.57 J1.3
!ACCEL_CS  (via drill 0.25)
  Top 0.203: 34.11,26.11 U2.22
  Top 0.254: 34.11,26.11 v34.54,26.54 | J5.7 v32,38.61
  Bottom 0.254: U5.9 35.86,25.36 34.67,26.54 | v34.54,26.54 34.67,26.54 | 34.67,26.54 34.67,35.94 v32,38.61
!OBS_CS  (via drill 0.25)
  Top 0.203: J6.8 19.81,47.75 20.83,46.74 20.83,45.72 19.49,44.39 8.32,44.39 6.6,42.67 6.6,27.43 7.49,26.54 10.23,26.54 J2.8 10.74,26.04
  Top 0.254: 10.92,25.65 J2.8 12.13,26.67 v12.19,26.67
  Bottom 0.254: U5.28 20.97,29.36 20.45,28.83 20.45,28.45 17.65,25.65 J1.8 16.32,26.67 v12.19,26.67
  Bottom 0.406: J6.8 19.81,51.05 J7.1
!PRESSURE_CS  (via drill 0.25)
  Top 0.254: v24.64,31.75 26.92,31.75 27.94,30.73 27.94,29.72 27.42,29.2 U1.8 | J5.15 v21.84,38.61
  Bottom 0.254: U5.20 26.49,24.31 24.64,26.16 v24.64,31.75 24.64,35.81 v21.84,38.61
!RESET
  Bottom 0.254: J3.6 19.3,39.75 19.3,40.64 18.54,41.4 17.53,41.4 16.76,40.64 16.76,36.83 16.51,36.58 16.51,35.05 20.21,31.36 U5.30
ACCEL_INT  (via drill 0.25)
  Top 0.203: U2.12 32.91,32.26 | 32.91,32.37 J5.8
  Top 0.254: 32.91,32.37 32.91,32.26 33.42,31.75 v35.56,31.75
  Bottom 0.254: v35.56,31.75 35.56,27.69 36.83,26.42 40.21,26.42 U5.8
BATTERY  (via drill 0.25)
  Top 0.254: 14.99,11.18 13.98,10.17 U10.8 | 13.46,12.95 v14.99,12.95 14.99,11.18 | 13.46,12.95 11.43,12.95 11.18,12.7 U10.1 | U10.12 13.08,12.57 13.46,12.95 | U10.10 14.99,11.18
  Top 0.406: C19.1 v20.32,11.68
  Bottom 0.406: J8.2 39.35,14.21 35.31,9.91 22.1,9.91 v20.32,11.68 19.05,12.95 v14.99,12.95
BBB_GPIO  (via drill 0.25)
  Top 0.203: J6.7 19.81,45.47 19.56,45.21 8.64,45.21 6.1,42.67 6.1,27.05 v6.6,26.54
  Top 0.254: J2.7 v14.22,25.65
  Bottom 0.203: J1.7 10.74,26.04 10.61,25.91 10.16,25.91 | 9.78,26.04 9.91,25.91 10.16,25.91 | v6.6,26.54 9.53,26.54 10.16,25.91
  Bottom 0.254: v14.22,25.65 J1.7
BBB_INT  (via drill 0.25)
  Top 0.254: v14.22,29.21 12.13,29.21 J2.10
  Bottom 0.254: v14.22,29.21 16.32,29.21 J1.10 18.8,28.19 20.96,30.36 U5.29
BBB_MISO  (via drill 0.2, 0.25)
  Top 0.203: J2.4 10.48,21.21 6.48,21.21 v6.1,21.59
  Top 0.254: J2.4 11.43,20.57 12.7,19.3 v14.22,19.3
  Bottom 0.203: J6.4 14.73,47.75 15.75,46.74 15.75,45.72 14.73,44.7 8.13,44.7 6.1,42.67 6.1,34.8 | P9/P8.P9_21 2.79,32.51 4.06,33.78 5.08,33.78 6.1,34.8 | v6.1,21.59 6.1,26.16 5.84,26.42 5.84,26.67 6.1,26.92 6.1,34.8
  Bottom 0.254: U5.26 21.13,27.36 20.07,26.29 20.07,21.72 18.92,20.57 J1.4 16.06,19.3 v14.22,19.3
BBB_MOSI  (via drill 0.2, 0.25)
  Top 0.203: J6.2 11.18,48.77 6.1,43.69 4.06,43.69 3.05,42.67 3.05,38.86 | v2.79,23.62 2.79,24.13 3.05,24.38 3.05,38.86 | P9/P8.P9_18 4.32,37.59 3.05,38.86 | J2.2 9.65,18.03 9.14,18.54 3.81,18.54 3.3,19.05 3.3,20.57 3.05,20.83 v3.05,21.08
  Top 0.254: J2.2 11.43,18.03 12.7,16.76 v14.22,16.76
  Bottom 0.203: v2.79,23.62 2.79,23.11 3.05,22.86 v3.05,21.08
  Bottom 0.254: U5.25 20.89,26.36 20.57,26.04 20.57,20.32 18.29,18.03 J1.2 16.06,16.76 v14.22,16.76
BBB_SCLK  (via drill 0.25)
  Top 0.203: 12.13,24.13 12.13,24.07 11.18,23.11 | 5.59,31.5 P9/P8.P9_22 | J6.6 16.26,47.75 10.67,47.75 5.59,42.67 5.59,31.5 | 10.86,23.37 J2.6 10.35,23.88 6.35,23.88 5.59,24.64 5.59,31.5
  Top 0.254: J2.6 12.13,24.13 v14.22,24.13
  Bottom 0.254: U5.27 21.12,28.36 19.56,26.8 19.56,24.51 18.29,23.24 18.29,23.11 J1.6 16.32,24.13 v14.22,24.13
BTLDR_CTRL  (via drill 0.25)
  Top 0.254: v21.34,24.38 19.81,25.91 19.81,31.75 16.51,35.05 16.51,37.34 v17.78,38.61
  Bottom 0.254: U5.24 21.34,24.98 v21.34,24.38 | v17.78,38.61 18.29,39.12 J3.5
BTLDR_RX
  Bottom 0.254: U5.22 24.49,24.28 23.37,25.4 23.37,34.42 J3.4
BTLDR_TX
  Bottom 0.254: J3.3 17.02,36.2 17.02,35.31 18.03,34.29 22.35,34.29 22.86,33.78 22.86,24.89 23.49,24.26 U5.23
EEPROM_SCL  (via drill 0.2)
  Top 0.203: 7.69,55.88 U7.SCL | 7.68,56.13 U7.SCL | v5.33,51.56 5.59,51.56 6.1,52.07 6.1,55.37 6.6,55.88 7.43,55.88 U7.SCL
  Bottom 0.203: P9/P8.P9_19 3.05,36.07 3.05,50.29 4.32,51.56 v5.33,51.56
EEPROM_SDA  (via drill 0.2)
  Top 0.203: U7.SDA 7.44,57.4 6.86,57.4 5.59,56.13 5.59,54.61 5.08,54.1 v3.3,54.1
  Bottom 0.203: P9/P8.P9_20 3.3,33.78 1.52,33.78 0.76,34.54 0.76,53.34 1.52,54.1 v3.3,54.1
GND  (via drill 0.25)
  Top 0.203: U2.11 33.31,30.52 33.58,30.79 | U2.18 32.77,26.21 33.1,26.34 | P9/P8.P9_44 4.57,5.08 | U10.3 11.88,11.17 U10.NC | 6.86,14.99 9.65,14.99 | 6.86,15.88 9.65,15.88
  Top 0.254: U4.2 30.86,3.17 31.24,3.56 31.24,4.45 30.99,4.7 30.23,4.7 29.34,5.59 29.34,7.24 | J2.9 v14.22,28.19 | 33.58,30.79 C4.2 | U1.5 27.04,26.94 v27.3,26.67 | U1.12 25.54,29.33 25.65,29.21 | U3.8 35.95,17.66 35.81,17.53 | U10.4 v10.16,10.67 10.66,11.17 U10.3 | U10.4 | U10.4 12.19,10.67 | U10.9 12.13,10.67 U10.NC | U10.11 12.19,11.67 12.19,11.68
  Top 0.406: U7.VSS 14.98,57.28 C12.2 | U9.GND 46.99,19.3 47.83,18.47 | U8.2 33.27,14.22 v32.51,14.99
  Bottom 0.203: 6.48,27.43 9.14,27.43 9.65,26.92 | 6.79,19.43 9.46,19.43
  Bottom 0.254: v14.22,28.19 J1.9 | J3.2 20.07,36.58 20.83,35.81
  other vias: 26.42,28.45 42.42,29.97 37.21,27.37 31.24,26.16 20.32,33.53 26.42,36.32 21.34,35.31 15.75,30.99 29.53,7.37 35.94,15.24 12.19,30.99 23.37,2.54 34.8,2.03 40.64,23.11 25.4,21.84 32.26,35.81 37.85,35.81 21.34,22.86 17.91,19.43 34.16,17.4 6.86,49.78 20.57,59.18 7.37,58.93 47.62,24.89 46.16,26.73 14.22,22.1 7.87,42.42 5.84,13.46 44.07,16.26 37.97,10.16 41.78,10.16 47.62,23.11 25.15,47.5 14.22,14.99 25.4,17.53 37.59,31.5 14.1,12.06 35.43,8.64
  pour Bottom: 49.53,1.02 33.53,1.02 33.53,6.86 24.64,6.86 24.64,1.02 8.64,1.02 8.61,37.87 arc-90 12.93,41.91 49.53,41.91
  pour Top: 49.53,1.02 33.53,1.02 33.53,6.86 24.64,6.86 24.64,1.02 8.64,1.02 8.61,37.62 arc-90 12.93,41.91 49.53,41.91
  pour Bottom: 27.94,43.18 12.19,43.18 arc90 7.37,38.35 7.62,0 0,0 0,60.45 27.94,60.45
  pour Top: 27.94,43.18 12.19,43.18 arc90 7.37,38.35 7.62,0 0,0 0,60.45 27.94,60.45
LIGHT_INT  (via drill 0.25)
  Top 0.254: J5.13 v24.38,38.61 | v38.35,19.81 38.54,19.62 U3.4 | R11.1 36.4,23.44 v34.04,21.08
  Bottom 0.254: v24.38,38.61 25.27,37.72 25.27,26.54 27.49,24.33 U5.19 27.49,22.04 28.45,21.08 v34.04,21.08 37.08,21.08 v38.35,19.81
MIC_AIN  (via drill 0.25)  (1 unrouted)
  Top 0.254: R10.2 v34.29,12.19 | v46.79,22.09 46.79,21.11
  Top 0.406: C1.1 34.04,11.18 33.53,11.68 33.53,12.12 R10.2 33.45,12.91 U8.1
  Bottom 0.254: v34.29,12.19 37.66,15.56 42.04,15.56 43.05,16.64 43.05,19.56 44.12,20.75 45.45,22.09 v46.79,22.09
MIC_INT
  Top 0.254: 43.69,20.34 U9.ALRT 43.76,20.26 43.76,20.83 R4.1
MISO  (via drill 0.25)
  Top 0.203: U2.9 34.11,28.01
  Top 0.254: 34.11,28.01 v33.66,27.56 | v29.84,35.31 29.84,33.66 J5.10 29.46,30.48 27.69,28.7 U1.7
  Bottom 0.254: U5.14 34.49,24.44 33.66,25.27 v33.66,27.56 33.66,31.5 v29.84,35.31
MOSI  (via drill 0.25)
  Top 0.203: 34.91,25 U2.24
  Top 0.254: 34.91,25 33.53,23.62 v33.53,22.23 | J5.9 v29.46,38.61 | U1.6 27.82,28.2 28.45,28.83 v29.97,28.83
  Bottom 0.254: v33.53,22.23 33.53,23.54 U5.15 33.49,24.17 32.77,24.89 31.5,24.89 29.97,26.42 v29.97,28.83 29.97,34.04 28.96,35.05 28.96,38.1 v29.46,38.61
N$1  (via drill 0.25)
  Top 0.406: v30.73,12.19 30.73,11.25 R3.1 C13.2
  Bottom 0.406: Q1.+ 28.42,19.59 30.73,16.76 v30.73,12.19
N$3
  Top 0.203: C4.1 33.71,29.74 U2.10
N$4
  Top 0.254: 36.7,16.64 36.7,17.1 U3.9
  Top 0.406: D1.CATHODE 36.7,16.64
N$5
  Top 0.254: C13.1 32.69,10.16 R66.1
N$6
  Top 0.254: 36.64,19.24 U3.6
  Top 0.406: D2.CATHODE 36.64,21.53 36.64,19.24
N$7  (via drill 0.25)
  Top 0.254: 35.68,18.16 U3.7
  Top 0.406: v32.26,9.14 34.04,9.14 35.05,10.16 35.05,17.53 35.68,18.16 | D3.CATHODE 18.67,3.93 v20.57,5.84
  Bottom 0.406: v32.26,9.14 23.88,9.14 v20.57,5.84
N$8  (via drill 0.25)
  Top 0.406: v31.5,8.13 33.78,8.13 35.31,6.6 35.31,3.05 36.32,2.03 38.61,2.03 39.5,2.92 D1.ANODE 39.61,3.67 C17.POS 39.61,15.73 40.72,16.84 R2.1 40.72,20.38 D2.ANODE | v22.1,5.84 21.47,5.21 D3.ANODE
  Bottom 0.406: v31.5,8.13 24.38,8.13 v22.1,5.84
N$9
  Top 0.254: 33.89,10.23 C1.2 33.83,10.23 32.97,11.1 R66.2 32.59,11.28 R10.1
  Top 0.406: R10.1 32.59,13.8 U8.4
N$10
  Top 0.254: U8.3 33.35,15.64 C14.1 33.27,16.26 32.33,17.2 R9.2 31.68,17.12 R8.1
N$11
  Top 0.254: R1.2 47.68,20.66 47.33,20.31
  Top 0.406: U9.VIN 46.48,20.31 47.33,20.31 C2.1
N$12  (via drill 0.25)
  Top 0.203: v17.02,6.86 17.03,6.85
  Top 0.254: 17.03,6.85 L1.1 | U10.2 11.18,11.68 v10.16,11.68
  Bottom 0.254: v17.02,6.86 12.19,11.68 v10.16,11.68
N$14  (via drill 0.25)
  Top 0.254: U11.P$1 45.65,11.24 44.96,11.94 v44.96,15.11 | R3.2 31.75,11.25 v31.75,12.19 31.75,12.74 U8.5 31.21,13.37 30.29,14.29 30.29,15.74 C10.1 R8.2
  Bottom 0.254: v44.96,15.11 38.48,15.11 34.54,11.18 32.77,11.18 v31.75,12.19
N$31
  Top 0.406: U7.WP 7.68,54.61 8.64,54.61 10.92,52.32 14.22,52.32 14.99,53.09 R5.2 15.35,53.45 17.27,55.37 J4.1
NAME  (via drill 0.2)
  other vias: 6.35,45.72
OBSERVER_INT
  Top 0.203: J6.10 22.35,49.53 22.1,49.78 11.68,49.78 6.1,44.2 3.56,44.2 P9/P8.P9_13
OPAMP_GATE  (via drill 0.25)
  Top 0.254: U11.P$3 48.19,13.14 v48.51,13.46 | J5.4 38.1,33.27 38.61,32.77 v38.61,29.46
  Bottom 0.254: v48.51,13.46 48.9,13.97 48.9,22.86 47.88,24.13 43.94,24.13 42.67,25.15 42.67,27.69 42.26,28.36 U5.6 39.46,28.36 v38.61,29.46
PIR_OUT  (via drill 0.25)
  Top 0.254: v34.54,38.61 J5.5 | v41.91,27.43 45.59,27.43 U6.OUT
  Bottom 0.254: v34.54,38.61 36.58,36.58 36.58,29.21 38.43,27.36 U5.7 41.83,27.36 v41.91,27.43
PRESSURE_INT  (via drill 0.25)
  Top 0.254: U1.11 26.04,30.61 25.65,30.99 v24,30.99 | v23.75,35.31 21.84,33.4 J5.16
  Bottom 0.254: U5.21 25.49,24.3 24,25.78 v24,30.99 24,35.05 v23.75,35.31
SCL  (via drill 0.25)
  Top 0.254: U4.6 26.78,2.17 26.29,2.67 26.29,4.83 26.67,5.21 27.81,5.21 28.32,5.71 28.32,23.24 28.83,23.75 | R7.1 29.97,26.16 v28.83,25.02 28.83,23.75 | J5.11 v26.92,38.61 | 28.83,23.75 33.27,19.3 v35.31,19.3 | v39.62,17.27 39.24,17.66 U3.2 | U9.SCL 43.43,19.3 41.66,17.53 v41.66,17.27
  Bottom 0.254: U5.17 29.49,24.36 v28.83,25.02 28.19,25.65 28.19,33.91 27.3,34.8 27.3,38.23 v26.92,38.61 | v35.31,19.3 37.34,17.27 v39.62,17.27 v41.66,17.27
SCLK  (via drill 0.25)
  Top 0.203: 34.51,25.24 U2.23
  Top 0.254: 34.51,25.24 34.29,25.02 31.11,25.02 v30.61,24.51 | J5.12 26.92,34.04 v27.94,35.05 | U1.4 26.54,26.55 27.05,26.04 27.69,26.04 28.19,26.54 28.19,27.43 28.7,27.94 v29.21,27.94
  Bottom 0.254: U5.16 31.54,23.58 v30.61,24.51 29.21,25.91 v29.21,27.94 29.21,33.78 v27.94,35.05
SDA  (via drill 0.25)
  Top 0.254: U4.1 31.26,2.17 31.75,2.67 31.75,4.83 31.37,5.21 30.35,5.21 29.84,5.71 29.84,6.73 30.23,7.11 30.23,7.75 29.84,8.13 29.84,20.95 | J5.14 24.38,33.4 v26.04,35.05 | v27.94,24.89 27.94,25.22 R6.1 | 29.84,20.95 v28.96,21.84 | v34.54,18.54 32.26,18.54 29.84,20.95 | v38.35,16.26 38.54,16.44 U3.1 | U9.SDA 43.75,18.35 v41.66,16.26
  Bottom 0.254: v26.04,35.05 25.78,34.8 25.78,27.05 v27.94,24.89 28.49,24.34 U5.18 28.49,22.31 v28.96,21.84 | v34.54,18.54 36.83,16.26 v38.35,16.26 v41.66,16.26
VCC  (via drill 0.2, 0.25)  (1 unrouted)
  Top 0.203: C8.1 34.51,29.25 U2.8 | 2.03,55.24 P9/P8.P9_3 0.76,54.1 0.76,16.76 1.52,16 v5.08,16
  Top 0.254: U4.5 27.3,3.17 26.92,3.56 26.92,4.45 27.18,4.7 27.94,4.7 28.83,5.59 28.83,20.19 v28.96,20.32 | C6.1 25.04,26.25 U1.1 24.31,27.5 24.07,27.75 23.55,28.27 C16.1 | U1.15 24.26,28.7 | 24.26,28.7 23.8,28.7 C16.1 | C16.1 C7.1 | U1.14 24.76,29.2 24.26,28.7 | 35.42,26.16 U2.1 36.38,26.18 C3.1 36.4,29.03 v37.34,29.97 35.23,29.97 C8.1 | R2.2 41.58,18.62 v41.66,18.54 | C9.1 39.62,19 v39.62,18.16 U3.3 | C5.1 32.06,28.52 U2.13 | 30.81,18.21 v30.73,18.29 | U10.5 10.68,10.17 9.91,9.4 | v10.16,13.46 9.4,12.7 9.4,9.91 9.91,9.4 | U11.P$2 46.09,16.88 46.99,17.53 | 9.91,9.4 10.16,9.14 17.78,9.14 18.54,9.91 | C20.1 18.29,10.16 18.54,9.91 | 18.54,9.91 18.8,9.65 18.8,8.71 L1.2 | R11.2 40.89,24.31 41.58,23.37
  Top 0.406: R6.2 R7.2 30.73,27.74 | 30.73,37.34 30.73,27.74 | 22.35,27.3 23.62,27.3 24.07,27.75 | 30.73,27.74 31.04,28.04 31.04,28.07 C5.1 | R2.2 41.58,23.37 41.58,23.42 U6.VCC 45.39,24.33 R4.2 | P9/P8.P9_4 P9/P8.P9_3 | R5.1 C12.1 14.97,56.01 U7.A2 12.63,55.88 11.68,55.88 11.18,55.37 v10.16,55.37 | U7.VCC 7.56,53.28 v6.86,52.58 | 45.47,21.52 45.47,18.8 45.91,18.35 U9.VA 46.42,17.84 46.74,17.53 46.99,17.53 48.69,17.53 | 48.69,17.53 C15.1 | 48.69,17.53 C11.1
  Top 0.61: v14.22,18.03 J2.1 18.29,18.03 v22.35,22.1 22.35,27.3 21.46,27.3 20.57,28.19 20.57,32.13 17.78,34.92 v17.78,35.81 19.3,37.34 30.73,37.34 38.86,37.34 39.62,38.1 v39.62,38.61 J5.1
  Bottom 0.203: J1.1 11.18,17.97 11.18,17.53 10.16,16.76 5.84,16.76 v5.08,16
  Bottom 0.254: v14.22,18.03 J1.1 | U5.1 38.94,33.35 38.61,33.02 38.61,31.24 v37.34,29.97 | v41.66,18.54 41.27,18.16 v39.62,18.16 | v30.73,18.29 30.73,19.3 29.84,20.19 29.08,20.19 v28.96,20.32 | v10.16,13.46 11.18,14.48 11.18,17.53
  Bottom 0.406: U5.1 44.37,33.35 47.75,29.97 47.75,26.92 46.61,25.78 U6.VCC | P9/P8.P9_4 6.1,55.37 | 6.1,55.37 v10.16,55.37 | 6.1,55.37 5.84,55.12 5.84,52.83 6.1,52.58 v6.86,52.58 6.86,51.56 J6.1
  Bottom 0.61: U5.1 40.27,37.97 v39.62,38.61 | v17.78,35.81 18.54,36.58 J3.1 | v28.96,20.32 24.13,20.32 v22.35,22.1
VDD
  Top 0.406: P9/P8.P9_6 P9/P8.P9_5

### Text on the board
tPlace: Observer | B. Campbell / N. Jackson / C. Kreng / A. Zhen | 2016/02/01 | X | Y | Z | Observer | D | B. Campbell / N. Jackson / C. Kreng / A. Zhen | 2016/02/01
tNames: EEPROM / WRITE | CHIPSELECT

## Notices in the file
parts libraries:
SparkFun-Passives: Licensing: CC v3.0 Share-Alike You are welcome to use this library for commercial purposes.
SparkFun-Aesthetics: Licensing: Creative Commons ShareAlike 4.0 International - https://creativecommons.org/licenses/by-sa/4.0
